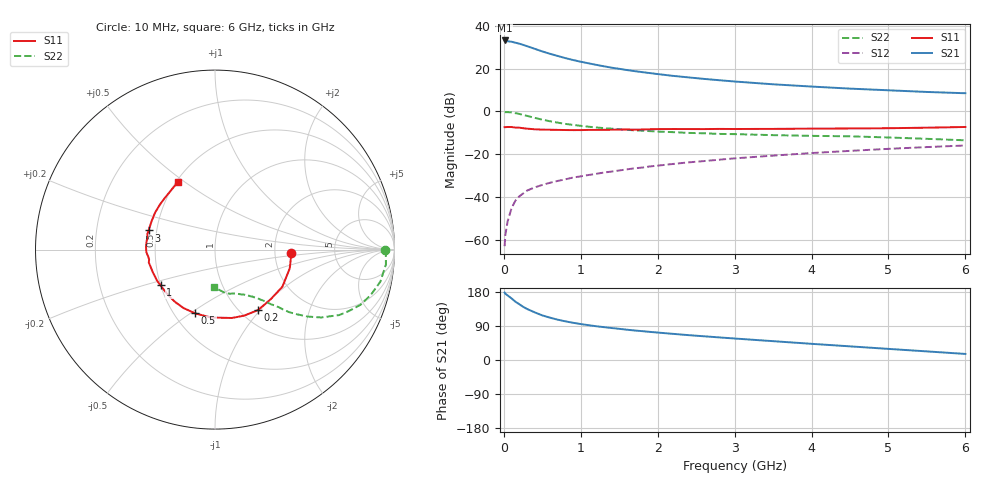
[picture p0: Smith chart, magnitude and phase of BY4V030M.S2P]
! SIEMENS Small Signal Semiconductors
! BFY420
! Si NPN RF SIEGET Grounded Emitter Transistor in MICRO-X
! VCE = 4 V  IC = 30 mA
! Common Emitter S-Parameters:  October  1996
# GHz  S  MA  R  50
!  f  S11  S21  S12  S22
! GHz  MAG  ANG  MAG  ANG  MAG  ANG  MAG  ANG
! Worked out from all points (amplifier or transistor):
!   36 points, 10 MHz to 6 GHz, reference 50 ohm
!   highest |S21| = 33.1 dB at 10 MHz (marker M1)
!   |S21| within 3 dB of that: start of sweep to 327.4 MHz
!   unconditionally stable (mu >= 1): start of sweep to 14.33 MHz; 1.695 GHz to end of sweep
!   at 250 MHz: K = 0.37, MSG = 34.8 dB, |S12| = -38.5 dB
!   at 1.4 GHz: K = 0.96, MSG = 24.3 dB, |S12| = -28.2 dB
!   at 6 GHz: K = 1.06, MAG = 10.8 dB, |S12| = -16.0 dB
!   S11 on the Smith chart (normalised r, x): 10 MHz: 2.48, -0.11; 200 MHz: 1.20, -0.97; 500 MHz: 0.63, -0.52; 1 GHz: 0.50, -0.23; 3 GHz: 0.45, +0.11; 6 GHz: 0.51, +0.47
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0.01  0.4259 -2.4  45.31 177.9  0.0007 91.2  0.9454 -0.1
0.02  0.4255 -5.5  44.89 174.9  0.0013 82.6  0.952 -1.3
0.1  0.4286 -28.9  42.28 162.6  0.0054 74.6  0.9383 -11.0
0.15  0.4158 -41.6  40.18 153.9  0.0081 72.5  0.9048 -16.1
0.2  0.4137 -54.7  38.17 147.4  0.0102 71.4  0.8679 -20.7
0.25  0.402 -66.3  35.72 140.5  0.0119 68.5  0.8225 -24.5
0.3  0.3925 -76.1  33.34 134.9  0.0139 66.5  0.7823 -27.8
0.4  0.3791 -93.4  28.97 125.8  0.0166 64.4  0.7019 -32.6
0.5  0.372 -107.2  25.08 117.7  0.0189 63.0  0.6361 -35.9
0.6  0.3699 -118.2  22.12 111.7  0.0213 62.5  0.5835 -38.2
0.7  0.3669 -127.3  19.66 106.4  0.0235 62.8  0.5421 -40.1
0.8  0.3642 -135.1  17.5 102.0  0.0256 61.8  0.5064 -41.3
1  0.3627 -146.8  14.4 94.9  0.0301 63.2  0.4566 -43.1
1.1  0.3664 -151.8  13.25 91.9  0.0323 63.2  0.4361 -44.3
1.4  0.3702 -163.3  10.47 84.4  0.0389 63.9  0.3921 -46.5
1.6  0.3758 -168.9  9.211 79.9  0.0438 62.9  0.3675 -48.3
2.2  0.3845 177.7  6.731 69.0  0.0586 61.2  0.3249 -53.0
3  0.385 163.9  4.97 56.7  0.0792 56.7  0.2922 -59.0
3.5  0.3872 155.8  4.275 49.7  0.0918 53.4  0.2765 -62.9
4.5  0.3963 140.8  3.387 36.0  0.1186 45.4  0.2593 -71.4
5.5  0.4131 125.5  2.83 22.7  0.1455 36.3  0.2267 -83.6
6  0.4292 119.0  2.641 16.0  0.1585 31.6  0.2092 -91.4
